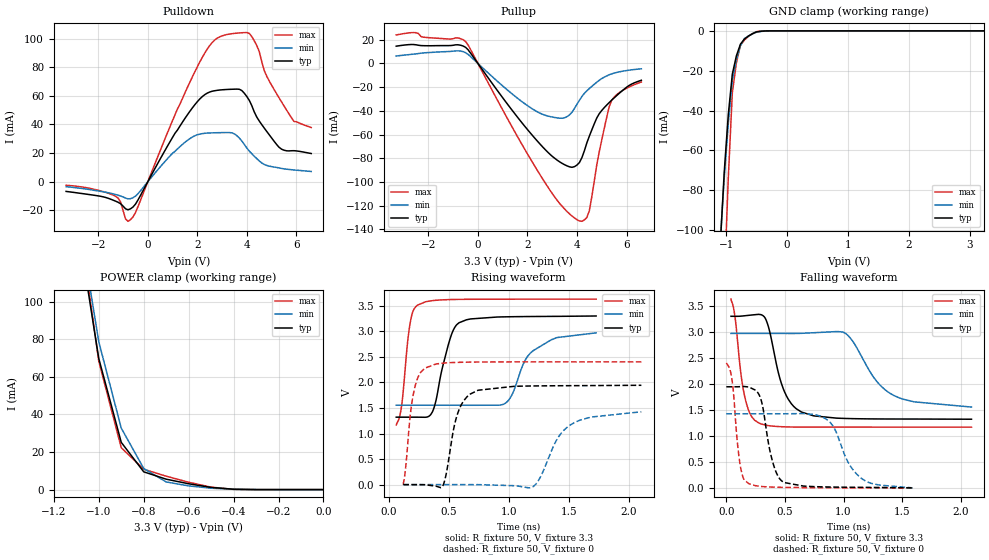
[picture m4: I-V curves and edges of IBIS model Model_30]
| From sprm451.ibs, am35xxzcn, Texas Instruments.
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| Model based on original model for BQ1833DV40DTPBFHP18LL_7LM
|   Sub model LL_7LM_PD_PU_OFF_3P3
[model]   Model_30
|[Description]  3.3V-I/O-PI-X
|[Input Load]   PI
|[Output Drive]
|Voltage   3.3V
|Mode   I/O
Model_type   I/O
Polarity   Non-Inverting
Enable   Active-Low
Vinl =  0.8V
Vinh =  2V
Cref =  15pF
Rref =  100.0000M
Vref =  0V
Vmeas =  1.65
C_comp   1.861386p   1.655853p   1.968812p
[Model Spec]
Vinl   0.8V   0.8V   0.8V
Vinh   2V   2V   2V
[Temperature Range]   25   125   -40
[Voltage Range]   3.3   2.97   3.63
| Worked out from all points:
|   slope of the pulldown table from 0 to 0.495 V, typ, clamps not added: 31.5 ohm
|   slope of the pullup table from 0 to 0.495 V, typ, clamps not added: 34.2 ohm
|   GND clamp passes 1 mA (typ) near -0.54 V on its own axis
|   POWER clamp passes 1 mA (typ) near -0.48 V on its own axis
|   rising waveform, R_fixture 50, V_fixture 3.3: 20-80 % time 118ps typ, 207ps min, 63.3ps max; typ from 1.32 V to 3.3 V
|   rising waveform, R_fixture 50, V_fixture 0: 20-80 % time 110ps typ, 206ps min, 72.2ps max; typ from 0 V to 1.94 V
|   falling waveform, R_fixture 50, V_fixture 3.3: 20-80 % time 145ps typ, 270ps min, 84.9ps max; typ from 3.3 V to 1.32 V
|   falling waveform, R_fixture 50, V_fixture 0: 20-80 % time 99.3ps typ, 182ps min, 58.3ps max; typ from 1.94 V to 0 V
[POWER_clamp]
-3.3V     2.432A     2.868A     2.62A
-1.067V   120.3mA    127.7mA    125.3mA
-1.033V   95.04mA    103.2mA    96.8mA
-1V       69.74mA    78.67mA    68.31mA
-900mV    25.15mA    32.72mA    22.27mA
-800mV    9.462mA    11.24mA    10.84mA
-700mV    5.548mA    4.085mA    7.139mA
-600mV    3.106mA    1.975mA    3.91mA
-500mV    1.161mA    745uA      1.301mA
-400mV    184uA      153.2uA    143uA
0V        9.359nA    44.03nA    36.65nA
[Pulldown]
-3.3V     -6.746mA   -3.451mA   -2.449mA
-1.3V     -13.56mA   -8.907mA   -10.16mA
-900mV    -18.87mA   -11.41mA   -25.91mA
-700mV    -18.91mA   -11.83mA   -26.47mA
2.1V      57.81mA    33.29mA    83.64mA
2.6V      63.23mA    34.14mA    97.21mA
3.2V      64.44mA    34.35mA    102.8mA
3.7V      64.57mA    30.45mA    103.9mA
4.1V      56.78mA    21.39mA    103.6mA
5.3V      24.08mA    9.65mA     58.63mA
5.9V      21.68mA    8.241mA    42.2mA
6.6V      19.7mA     7.18mA     37.87mA
[Pullup]
-3.3V     14.58mA    6.278mA    24.04mA
-2.5V     15.74mA    8.096mA    25.94mA
-500mV    13.62mA    9.123mA    18.54mA
1.5V      -42.71mA   -27.72mA   -58.1mA
2.6V      -70.12mA   -42.82mA   -96.98mA
3.5V      -85.45mA   -45.81mA   -122.9mA
4.1V      -83.57mA   -31.01mA   -132.9mA
4.4V      -66.93mA   -23.06mA   -130mA
4.5V      -61.28mA   -21.14mA   -124.2mA
4.9V      -42.37mA   -14.19mA   -74.57mA
5.4V      -31.02mA   -8.795mA   -31.2mA
6.6V      -14.18mA   -4.519mA   -15.68mA
[GND_clamp]
-3.3V     -2.048A    -1.805A    -3.667A
-1.1V     -108.6mA   -106.5mA   -191.4mA
-1.033V   -71.11mA   -74.03mA   -127.7mA
-966.7mV  -42.16mA   -46.82mA   -74.24mA
-900mV    -21.73mA   -24.87mA   -31.1mA
-833.3mV  -12.58mA   -14.46mA   -16.07mA
-766.7mV  -6.691mA   -7.462mA   -7.232mA
-700mV    -4.066mA   -3.873mA   -4.582mA
-566.7mV  -1.404mA   -1.475mA   -1.319mA
-500mV    -501.5uA   -687.7uA   -361.4uA
-300mV    -14.92uA   -26.13uA   -14.52uA
3.233V    8.845nA    14.35uA    33.57nA
[Ramp]
dV/dt_f  1.2101604/0.14626915n 0.87151911/0.27190974n  1.4966645/85.347181p
dV/dt_r  1.2019601/0.11117559n 0.89305234/0.20763443n  1.4662994/72.501172p
R_load = 50
[Rising Waveform]
R_fixture = 50
V_fixture = 3.3
V_fixture_min = 2.97
V_fixture_max = 3.63
64.02ps   1.32V      1.554V     1.168V
110.8ps   1.32V      1.554V     1.575V
181.4ps   1.32V      1.554V     3.18V
240.2ps   1.32V      1.554V     3.511V
368.7ps   1.443V     1.554V     3.601V
509.7ps   2.835V     1.553V     3.621V
586.6ps   3.168V     1.553V     3.625V
963.7ps   3.283V     1.581V     3.629V
1.192ns   3.29V      2.601V     3.63V
1.727ns   3.3V       2.97V      3.63V
[Rising Waveform]
R_fixture = 50
V_fixture = 0
V_fixture_min = 0
V_fixture_max = 0
123.1ps   8.59nV     120.6nV    4.064nV
204.2ps   177.1uV    1.777uV    1.743V
301.2ps   -2.104mV   2.583uV    2.279V
449.7ps   -31.91mV   -6.615uV   2.376V
577.5ps   1.408V     34.59uV    2.392V
745.4ps   1.847V     93.65uV    2.4V
1.19ns    1.931V     -54.64mV   2.402V
1.411ns   1.935V     924.4mV    2.402V
1.508ns   1.936V     1.162V     2.402V
2.103ns   1.944V     1.425V     2.402V
[Falling Waveform]
R_fixture = 50
V_fixture = 3.3
V_fixture_min = 2.97
V_fixture_max = 3.63
40ps      3.3V       2.97V      3.63V
73.14ps   3.3V       2.97V      3.3V
154.4ps   3.309V     2.97V      1.78V
276ps     3.337V     2.97V      1.249V
348.3ps   3.176V     2.97V      1.201V
495.8ps   1.852V     2.97V      1.174V
640.8ps   1.458V     2.972V     1.169V
1.015ns   1.335V     2.973V     1.169V
1.47ns    1.324V     1.735V     1.168V
2.092ns   1.32V      1.554V     1.168V
[Falling Waveform]
R_fixture = 50
V_fixture = 0
V_fixture_min = 0
V_fixture_max = 0
0s        1.944V     1.425V     2.402V
50.81ps   1.944V     1.425V     2.039V
121.2ps   1.947V     1.425V     398.3mV
192.3ps   1.94V      1.425V     79.35mV
290.9ps   1.729V     1.425V     28.53mV
400ps     462.3mV    1.425V     14.19mV
492.6ps   102.8mV    1.425V     9.235mV
867.6ps   17.14mV    1.297V     1.638mV
1.2ns     9.028mV    116.7mV    287uV
1.589ns   8.59nV     120.6nV    4.064nV
